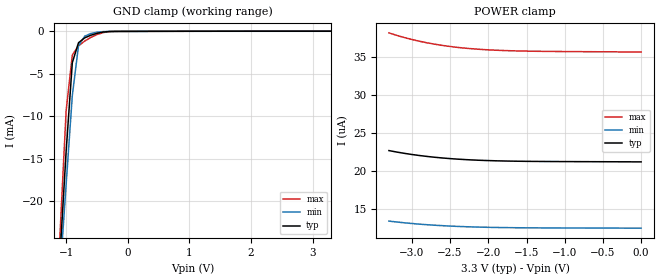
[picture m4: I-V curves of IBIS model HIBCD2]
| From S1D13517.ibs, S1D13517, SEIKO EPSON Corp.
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[Model]   HIBCD2
Model_type Input
C_comp   5p   4p   6p
[Temperature Range] 50   100   0
[Voltage Range]   3.3   3.0   3.6
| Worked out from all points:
|   GND clamp passes 1 mA (typ) near -0.74 V on its own axis
[GND Clamp]
-3.3V     -318.2mA   -279.4mA   -372.2mA
-1.1V     -26.39mA   -28.6mA    -23.95mA
-1V       -14.11mA   -18.01mA   -9.319mA
-900mV    -3.687mA   -7.551mA   -2.791mA
-800mV    -1.341mA   -1.706mA   -1.708mA
-700mV    -766.2uA   -575.6uA   -1.149mA
-600mV    -455.6uA   -251.6uA   -714.4uA
-500mV    -232.5uA   -98.77uA   -377.5uA
-300mV    -16.89uA   -5.974uA   -29.05uA
3.3V      21.2uA     12.48uA    35.65uA
[POWER Clamp]
-3.3V     22.69uA    13.4uA     38.19uA
-3.1V     22.33uA    13.18uA    37.58uA
-3V       22.18uA    13.09uA    37.32uA
-2.8V     21.92uA    12.93uA    36.88uA
-2.7V     21.81uA    12.86uA    36.7uA
-2.5V     21.64uA    12.75uA    36.4uA
-2.4V     21.57uA    12.71uA    36.28uA
-2.2V     21.45uA    12.64uA    36.09uA
-1.9V     21.35uA    12.57uA    35.91uA
-1.5V     21.28uA    12.52uA    35.79uA
-1.1V     21.25uA    12.5uA     35.74uA
0V        21.2uA     12.48uA    35.67uA
